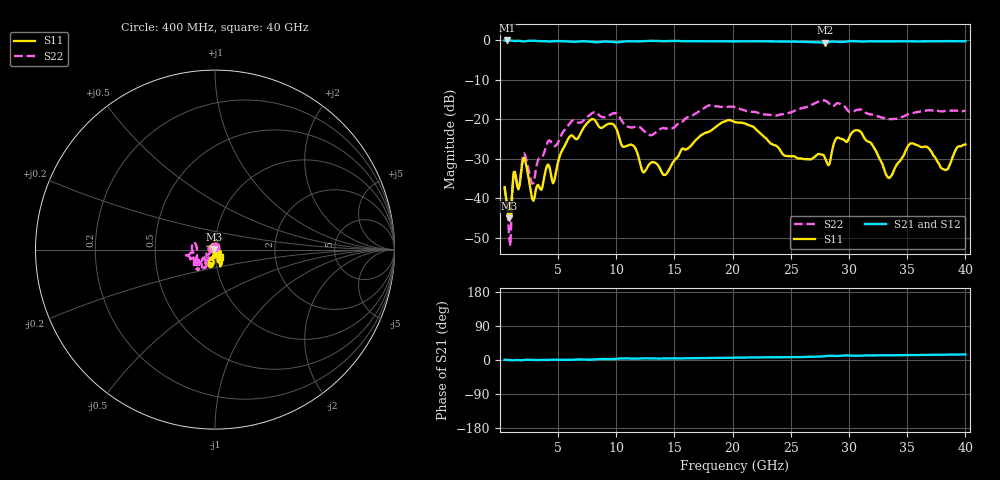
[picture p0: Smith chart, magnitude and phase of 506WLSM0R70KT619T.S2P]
!  American Technical Ceramics  Date:  8/31/2012
!  One Norden Lane
!  Huntington Station,  NY.  11746-2102
!  Tel:  (631) 622-4700  Fax:  (631) 622-4748
!  Part Number  506WLSM0R70KT619T
!  Description:  Ultra-Broadband Inductor
!  Application:  Ultra-broadband DC block decoupling, bias tee
# GHZ S DB R 50
! Freq  |S11|  S11 Ph  |S21|  S21 Ph  |S12|  S12 Ph  |S22|  S22 Ph
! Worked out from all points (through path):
!   401 points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, 400 MHz to 40 GHz, reference 50 ohm
!   highest |S21| = -0.01 dB at 598 MHz (marker M1); lowest = -0.5 dB at 27.92 GHz (marker M2)
!   lowest |S11| = -45.0 dB at 796 MHz (marker M3), VSWR 1.01, Z = 49.5 + j0.272 ohm
!   |S11| at or under -10 dB: start of sweep to end of sweep
!   |S22| runs from -52.1 to -15.2 dB; largest |S21 - S12| = 0.0039
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0.4  -37.15 105.5  -0.01 0.6  -0.01 0.6  -37.18 100.0
0.598  -41.59 117.5  -0.01 0.2  -0.01 0.2  -42.09 105.0
0.796  -45.05 150.6  -0.02 -0.1  -0.01 -0.1  -49.78 127.3
1.291  -33.37 156.8  -0.17 -0.1  -0.17 -0.1  -33.18 178.5
1.588  -37.74 162.3  -0.10 -0.2  -0.10 -0.3  -37.48 179.2
2.083  -29.75 148.5  -0.28 0.4  -0.28 0.4  -28.60 172.0
2.875  -40.65 159.9  -0.10 0.1  -0.09 0.1  -36.16 -171.4
4.162  -31.45 -156.2  -0.29 0.2  -0.29 0.2  -25.45 -148.4
4.657  -35.70 -126.1  -0.19 1.0  -0.19 0.9  -26.77 -149.0
5.845  -25.04 -105.6  -0.25 0.3  -0.25 0.3  -21.63 -125.7
7.033  -22.96 -95.7  -0.23 1.4  -0.23 1.3  -20.67 -123.9
9.607  -21.13 -107.7  -0.36 2.3  -0.37 2.3  -18.66 -118.9
12.28  -33.35 -83.9  -0.21 4.4  -0.22 4.4  -22.68 -141.6
13.666  -32.00 -72.0  -0.17 3.9  -0.17 3.9  -22.74 -143.3
20.2  -20.71 -71.1  -0.27 6.4  -0.27 6.5  -16.91 -131.6
26.833  -29.96 -60.5  -0.41 8.4  -0.42 8.5  -16.24 -167.4
27.922  -29.69 -88.4  -0.55 10.2  -0.55 10.3  -15.23 -167.7
30.793  -22.82 -60.3  -0.26 11.2  -0.25 11.3  -17.52 -145.1
33.466  -34.90 12.4  -0.25 12.4  -0.24 12.5  -19.92 -174.6
35.347  -26.08 78.0  -0.23 12.7  -0.24 12.8  -18.46 160.4
38.218  -32.76 5.3  -0.18 14.1  -0.17 14.2  -17.91 -171.6
40  -26.34 -55.1  -0.20 14.6  -0.20 14.7  -17.86 -146.4
